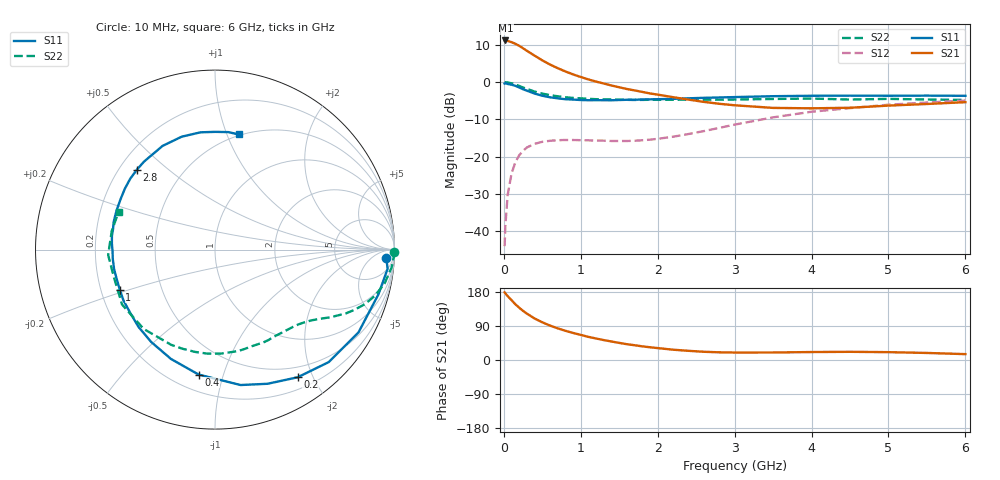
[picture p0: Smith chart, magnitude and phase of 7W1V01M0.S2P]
! Infineon Technologies  Discrete & RF Semiconductors
! BFS17W
! Si NPN RF Bipolar Junction Transistor in SOT323
! VCE = 1 V  IC = 1 mA
! Common Emitter S-Parameters:  August  1999
# GHz  S  MA  R  50
!  f  S11  S21  S12  S22
! GHz  MAG  ANG  MAG  ANG  MAG  ANG  MAG  ANG
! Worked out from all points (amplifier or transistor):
!   36 points, 10 MHz to 6 GHz, reference 50 ohm
!   highest |S21| = 11.2 dB at 20 MHz (marker M1)
!   |S21| within 3 dB of that: start of sweep to 316.9 MHz
!   unconditionally stable (mu >= 1): 954.5 MHz to end of sweep
!   at 250 MHz: K = 0.29, MSG = 13.8 dB, |S12| = -18.4 dB
!   at 1.4 GHz: K = 1.36, MAG = 3.8 dB, |S12| = -15.8 dB
!   at 6 GHz: K = 1.13, MAG = -2.4 dB, |S12| = -4.9 dB
!   S11 on the Smith chart (normalised r, x): 10 MHz: 20, -22; 200 MHz: 0.35, -1.78; 400 MHz: 0.30, -0.83; 1 GHz: 0.28, -0.19; 2.8 GHz: 0.27, +0.39; 6 GHz: 0.49, +1.10
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0.01  0.9566 -2.9  3.591 178.5  0.0063 86.3  0.9999 -0.7
0.02  0.9674 -6.4  3.621 175.5  0.012 85.4  0.9966 -2.3
0.05  0.9441 -15.3  3.566 168.5  0.0307 80.5  0.9889 -5.8
0.1  0.9231 -30.0  3.435 157.8  0.0594 72.3  0.9635 -11.3
0.15  0.8912 -44.7  3.266 147.1  0.0842 63.7  0.9275 -16.1
0.2  0.8473 -57.1  3.067 137.9  0.1046 57.5  0.8885 -20.0
0.25  0.8029 -68.6  2.844 129.6  0.1197 51.0  0.8459 -23.4
0.3  0.7679 -79.3  2.629 122.3  0.1329 46.5  0.8111 -26.0
0.4  0.702 -97.5  2.265 109.5  0.1486 38.4  0.7466 -30.3
0.5  0.6568 -111.9  1.957 99.5  0.1582 33.1  0.7019 -33.3
0.6  0.6258 -124.5  1.722 90.8  0.1634 29.5  0.6693 -36.0
0.8  0.5895 -143.3  1.391 77.1  0.1674 25.1  0.6271 -41.4
1  0.5755 -157.2  1.171 66.2  0.1664 23.7  0.6057 -46.6
1.1  0.5716 -163.8  1.086 61.0  0.1657 23.6  0.597 -49.8
1.6  0.5794 172.4  0.808 41.7  0.1623 29.5  0.5784 -66.0
2.2  0.5963 152.0  0.628 27.2  0.1852 43.1  0.5802 -86.8
2.8  0.6225 134.4  0.512 20.3  0.2432 50.4  0.5812 -108.2
3.5  0.6474 116.8  0.451 19.8  0.3368 49.2  0.5943 -131.9
4  0.6559 106.4  0.445 21.0  0.4004 44.1  0.6016 -149.4
4.5  0.6584 97.0  0.453 21.6  0.4478 38.3  0.5839 -164.7
5.5  0.6588 83.5  0.509 18.6  0.5325 27.1  0.5845 169.7
6  0.655 78.4  0.538 15.5  0.5658 21.8  0.5766 158.5
